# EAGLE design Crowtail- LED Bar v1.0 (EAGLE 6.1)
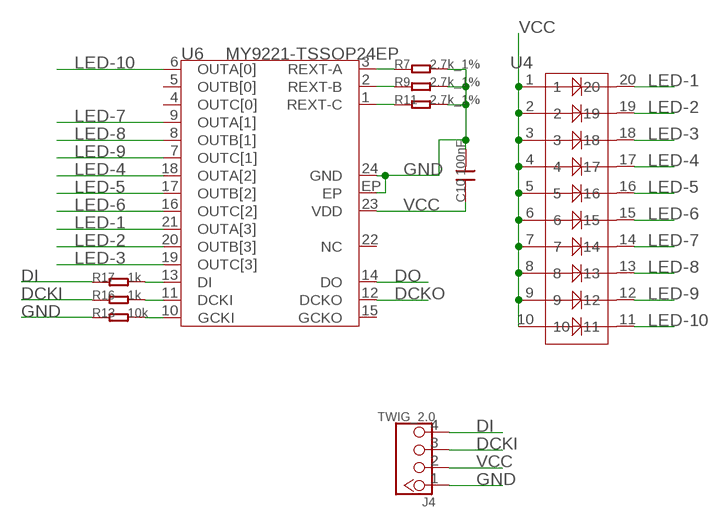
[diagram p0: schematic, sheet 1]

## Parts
C10  100nF  C-0603  [0603]
J4  TWIG_2.0  [2.0_1X4]
R7  2.7k_1%  R-0603  [0603]
R9  2.7k_1%  R-0603  [0603]
R11  2.7k_1%  R-0603  [0603]
R13  10k  R-0603  [0603]
R16  1k  R-0603  [0603]
R17  1k  R-0603  [0603]
U4  LED-20P  [20P-DIP-2.54-25.5X10.1X8.4H]
U6  MY9221-TSSOP24EP  [TSSOP24EP]

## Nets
DCKI: J4.3 R16.1
DCKO: U6.12(DCKO)
DI: J4.4 R17.1
DO: U6.14(DO)
GND: C10.2 J4.1 R7.2 R9.2 R11.2 R13.1 U6.24(GND) U6.EP
LED-1: U4.20 U6.21(OUTA[3])
LED-2: U4.19 U6.20(OUTB[3])
LED-3: U4.18 U6.19(OUTC[3])
LED-4: U4.17 U6.18(OUTA[2])
LED-5: U4.16 U6.17(OUTB[2])
LED-6: U4.15 U6.16(OUTC[2])
LED-7: U4.14 U6.9(OUTA[1])
LED-8: U4.13 U6.8(OUTB[1])
LED-9: U4.12 U6.7(OUTC[1])
LED-10: U4.11 U6.6(OUTA[0])
N$1: R17.2 U6.13(DI)
N$2: R16.2 U6.11(DCKI)
N$4: R13.2 U6.10(GCKI)
N$7: R11.1 U6.1(REXT-C)
N$8: R9.1 U6.2(REXT-B)
N$9: R7.1 U6.3(REXT-A)
VCC: C10.1 J4.2 U4.1 U4.2 U4.3 U4.4 U4.5 U4.6 U4.7 U4.8 U4.9 U4.10 U6.23(VDD)
Unconnected: U6.4(OUTC[0]) U6.5(OUTB[0]) U6.15(GCKO) U6.22(NC)

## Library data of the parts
C10 = Discrete:C*: Ceramic Capacitors
J4 = CONNECTER:TWIG_2.0
R7 R9 R11 R13 R16 R17 = Discrete:R*
U4 = Module:LED-20P
U6 = For_Test_Albert:MY9221

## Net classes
0 default: width 0.203 mm, drill 0.305 mm, clearance 0.152 mm

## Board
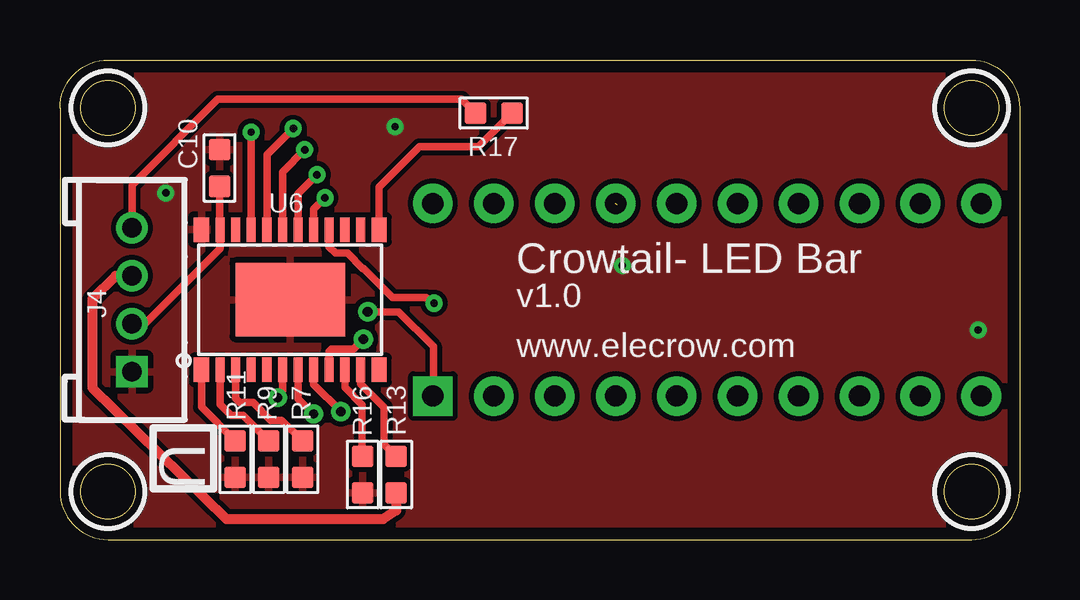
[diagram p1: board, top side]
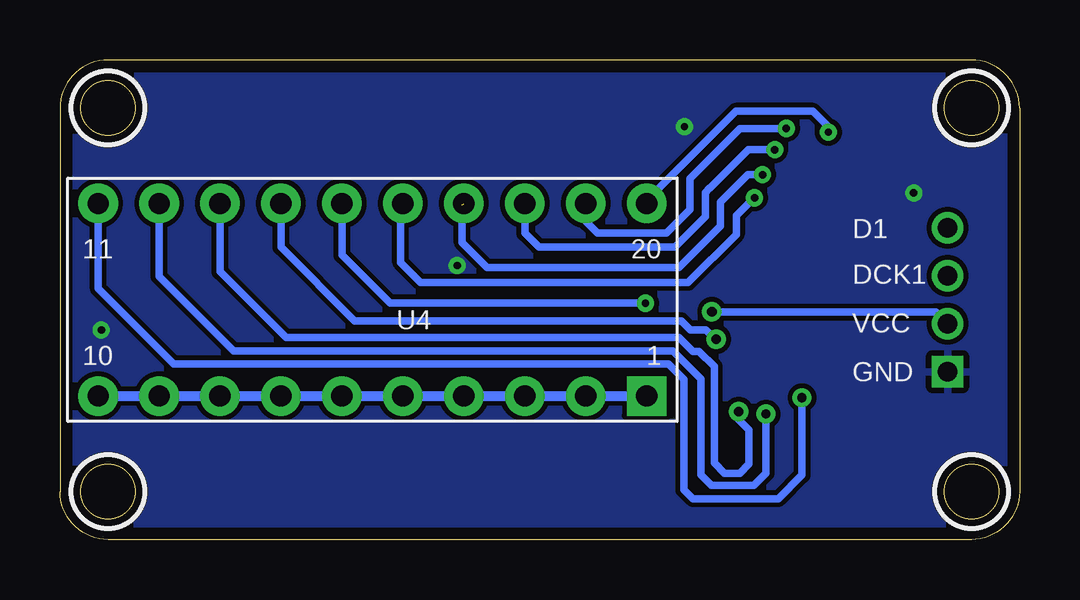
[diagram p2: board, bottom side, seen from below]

Size 40 x 20 mm. Coordinates in mm from the lower left corner, seen from the top.
Outline: 0,18 0,2 arc90 2,0 38,0 arc90 40,2 40,18 arc90 38,20 2,20 arc90 0,18
Outline: circle at 2,18 radius 1.14
Outline: circle at 2,18 radius 1.14
Outline: circle at 2,2 radius 1.14
Outline: circle at 38,18 radius 1.14
Outline: circle at 38,18 radius 1.14
Outline: circle at 38,2 radius 1.14
Outline: circle at 38,2 radius 1.14
Copper layers (1*16): Top 0.035mm / dielectric 1.5mm / Bottom 0.035mm
Design rules "default *": minimum track width 10mil, minimum drill 10mil, track to track 8mil, track to pad 8mil, pad to pad 8mil, via to via 8mil, smd to smd 8mil, copper to edge 20mil, drill to drill 8mil, minimum pad ring 10mil, minimum via ring 8mil, stop-mask expansion 4mil, vias tented up to drill 100mil, thermal gap 10mil
tRestrict: area 0.5,16.5 to 3.5,19.5; area 0.5,0.5 to 3.5,3.5; area 36.5,16.5 to 39.5,19.5; area 36.5,0.5 to 39.5,3.5
bRestrict: area 0.5,16.5 to 3.5,19.5; area 0.5,0.5 to 3.5,3.5; area 36.5,16.5 to 39.5,19.5; area 36.5,0.5 to 39.5,3.5

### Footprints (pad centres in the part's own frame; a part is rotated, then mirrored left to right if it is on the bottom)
0603 = smd 0.889 x 0.889: 1 -0.762,0; 2 0.762,0
2.0_1X4 = drill 0.8 pad 1.27 square: 1 -3,0 | drill 0.8 pad 1.27: 2 -1,0; 3 1,0; 4 3,0
20P-DIP-2.54-25.5X10.1X8.4H = drill 0.889 pad 1.651 square: 1 -11.43,4.013 | drill 0.889 pad 1.651: 2 -8.89,4.013; 3 -6.35,4.013; 4 -3.81,4.013; 5 -1.27,4.013; 6 1.27,4.013; 7 3.81,4.013; 8 6.35,4.013; 9 8.89,4.013; 10 11.43,4.013; 11 11.43,-4.013; 12 8.89,-4.013; 13 6.35,-4.013; 14 3.81,-4.013; 15 1.27,-4.013; 16 -1.27,-4.013; 17 -3.81,-4.013; 18 -6.35,-4.013; 19 -8.89,-4.013; 20 -11.43,-4.013
TSSOP24EP = smd 0.635 x 1.016: 1 -3.702,-2.921; 12 3.702,-2.921; 13 3.702,2.921; 24 -3.702,2.921 | smd 0.381 x 1.016: 2 -2.925,-2.921; 3 -2.275,-2.921; 4 -1.625,-2.921; 5 -0.975,-2.921; 6 -0.325,-2.921; 7 0.325,-2.921; 8 0.975,-2.921; 9 1.625,-2.921; 10 2.275,-2.921; 11 2.925,-2.921; 14 2.925,2.921; 15 2.275,2.921; 16 1.625,2.921; 17 0.975,2.921; 18 0.325,2.921; 19 -0.325,2.921; 20 -0.975,2.921; 21 -1.625,2.921; 22 -2.275,2.921; 23 -2.925,2.921 | smd 4.572 x 3.048: EP 0,0

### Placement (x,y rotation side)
C10  6.65,15.49 90 top
J4  3,10 90 top
R7  10.11,3.35 270 top
R9  8.71,3.35 270 top
R11  7.31,3.35 270 top
R13  12.62,2.71 90 top
R16  14.01,2.71 90 top
R17  18.08,17.78 0 top
U4  26.98,10 180 bottom
U6  9.6,10 0 top

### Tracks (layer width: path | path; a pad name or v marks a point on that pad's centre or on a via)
DCKI
  Top 0.406: J4.3 2.31,11 1.35,10.03 1.35,6.33 6.93,0.86 13.49,0.86 14.01,1.21 R16.1
DI
  Top 0.305: J4.4 3,14.79 6.58,18.36 16.74,18.36 R17.1
GND  (via drill 0.3)
  other vias: 23.44,11.43 4.41,14.45 13.96,17.22 38.27,8.74
  pour Top: -0.76,20.83 40.89,20.83 40.89,-0.64 -0.76,-0.64
  pour Bottom: -0.64,20.7 40.77,20.7 40.77,-0.51 -0.64,-0.51
LED-1  (via drill 0.3)
  Top 0.305: U6.21 v7.97,16.99
  Bottom 0.305: v7.97,16.99 7.97,17.22 8.61,17.86 11.83,17.86 15.41,14.28 15.41,14.15 U4.20
LED-2  (via drill 0.3)
  Top 0.305: U6.20 8.62,16.05 v9.72,17.14
  Bottom 0.305: U4.19 18.05,13.98 18.05,13.23 17.6,12.78 14.73,12.78 13.74,13.77 13.74,15.06 11.65,17.14 v9.72,17.14
LED-3  (via drill 0.3)
  Top 0.305: U6.19 9.28,15.32 v10.21,16.26
  Bottom 0.305: v10.21,16.26 11.3,16.26 12.9,14.66 12.92,14.66 13.1,14.48 13.1,13.46 14.37,12.19 20.04,12.19 20.62,12.78 U4.18
LED-4  (via drill 0.3)  (1 unrouted)
  Top 0.305: U6.18 9.93,14.43 v10.71,15.21
  Bottom 0.305: v10.71,15.21 11.32,15.21 12.47,14.07 12.47,13.08 14.19,11.35 22.2,11.35 23.24,12.39 23.24,13.94
LED-5  (via drill 0.3)
  Top 0.305: U6.17 10.57,13.78 v11.04,14.25
  Bottom 0.305: v11.04,14.25 11.07,14.25 11.81,13.51 11.81,12.72 13.81,10.72 24.96,10.72 25.8,11.56 25.8,13.87 25.71,13.96 U4.16
LED-6  (via drill 0.3)
  Top 0.305: U6.16 11.22,12.19 11.48,11.94 11.99,11.94 12.62,11.3 12.65,11.3 13.87,10.08 15.27,10.08 v15.6,9.86
  Bottom 0.305: U4.15 28.25,11.86 28.24,11.86 26.23,9.86 v15.6,9.86
LED-7  (via drill 0.41)
  Top 0.305: v12.65,8.36 12.24,7.95 11.33,7.95 11.22,7.85 U6.9
  Bottom 0.305: v12.65,8.36 12.7,8.36 13.08,8.74 13.72,8.74 14.1,9.12 27.71,9.12 30.79,12.19 U4.14
LED-8  (via drill 0.41)
  Top 0.305: U6.8 10.57,6.47 v11.71,5.33
  Bottom 0.305: v11.71,5.33 11.71,5 11.28,4.57 11.28,3.15 11.66,2.77 12.29,2.77 12.72,3.2 12.72,7.21 13.36,7.85 13.61,7.85 14.2,8.43 30.58,8.43 33.33,11.18 U4.13
LED-9  (via drill 0.38)
  Top 0.305: U6.7 9.93,5.87 v10.57,5.23
  Bottom 0.305: v10.57,5.23 10.57,2.77 11.07,2.26 12.85,2.26 13.28,2.69 13.28,6.71 14.45,7.87 32.77,7.87 35.87,10.97 U4.12
LED-10  (via drill 0.38)
  Top 0.305: U6.6 9.28,6.2 v9.07,5.92
  Bottom 0.305: U4.11 38.41,10.46 35.26,7.32 14.63,7.32 13.99,6.68 13.99,2.08 13.61,1.7 10.06,1.7 9.07,2.69 v9.07,5.92
N$1
  Top 0.305: U6.13 13.3,14.7 14.99,16.38 17.44,16.38 R17.2
N$2
  Top 0.305: U6.11 12.53,6.5 13.51,5.51 13.51,3.97 R16.2
N$4
  Top 0.305: U6.10 11.88,6.34 12.6,5.61 12.6,3.49 R13.2
N$7
  Top 0.305: U6.1 5.9,5.52 R11.1
N$8
  Top 0.305: U6.2 6.67,5.64 7.14,5.18 7.64,5.18 R9.1
N$9
  Top 0.305: U6.3 7.33,5.88 7.49,5.71 8.05,5.71 8.79,4.98 9.24,4.98 R7.1
VCC  (via drill 0.41)
  Top 0.305: J4.2 3.54,9 6.68,12.14 U6.23 6.65,12.94 C10.1 | v12.83,9.5 14.12,9.5 15.57,8.05 15.57,6.01 U4.1 | U4.4
  Bottom 0.305: v12.83,9.5 3.5,9.5 J4.2
  Bottom 0.406: U4.10 U4.9 U4.8 U4.7 U4.6 U4.5 U4.4 U4.3 U4.2 U4.1

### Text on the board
tPlace: Crowtail- LED Bar | v1.0 | www.elecrow.com | U
bPlace: D1 | DCK1 | VCC | GND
